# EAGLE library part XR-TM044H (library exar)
T1 REPEATER
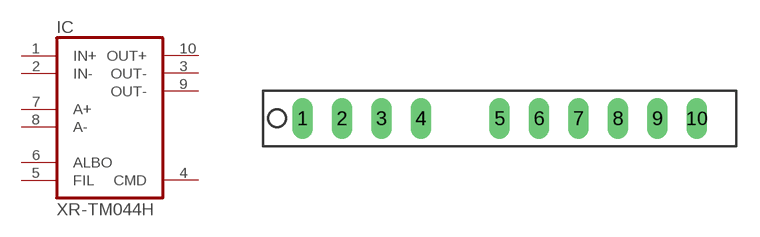
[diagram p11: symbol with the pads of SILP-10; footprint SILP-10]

Designator prefix IC

## XR-TM044H (OC_FARNELL: unknown; OC_NEWARK: unknown)  [SILP-10]
1  IN+  in
2  IN-  in
3  OUT-  out
4  CMD  pwr
5  FIL  in
6  ALBO  in
7  A+  in
8  A-  in
9  OUT-  out
10  OUT+  out

## Footprint SILP-10 (pad centres in mm)
Single Inline Package
drill 0.813 long: 1 -10.16,0; 2 -7.62,0; 3 -5.08,0; 4 -2.54,0; 5 2.54,0; 6 5.08,0; 7 7.62,0; 8 10.16,0; 9 12.7,0; 10 15.24,0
